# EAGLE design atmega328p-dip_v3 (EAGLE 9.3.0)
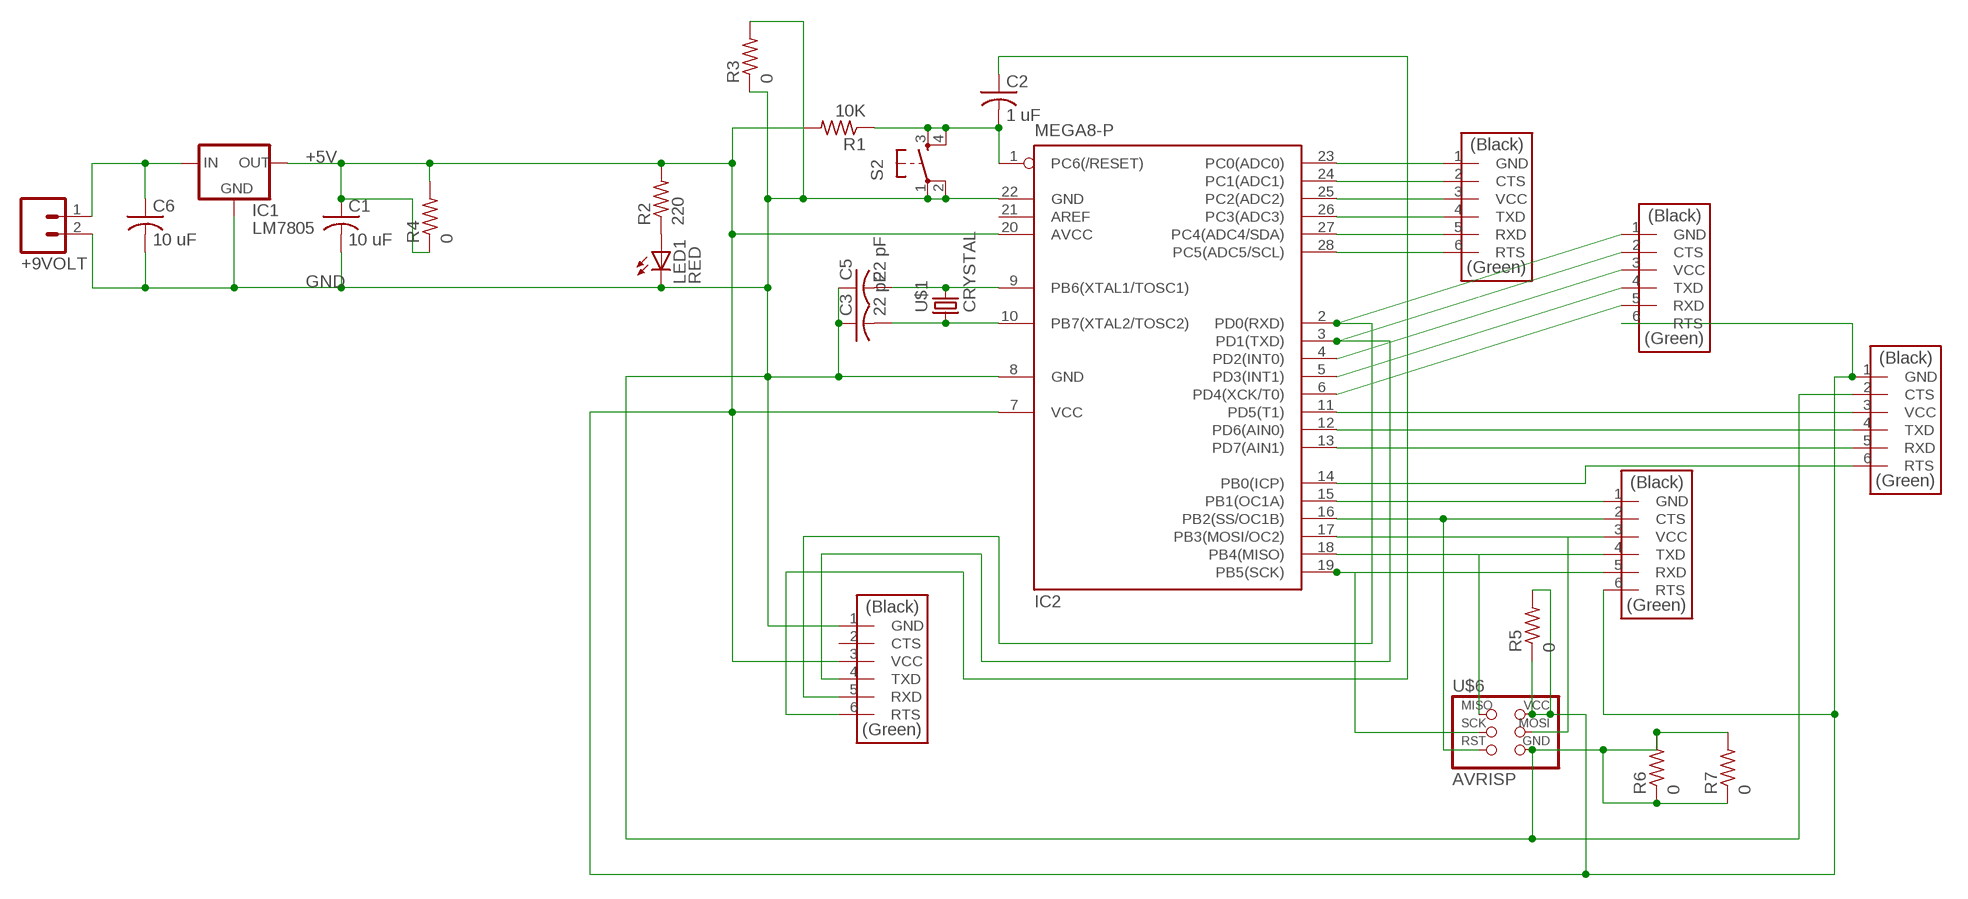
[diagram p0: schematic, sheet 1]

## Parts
+9VOLT  M02PTH4  [1X02_XTRA_BIG]
C1  10 uF  C-USC1206  [C1206]
C2  1 uF  C-USC1206  [C1206]
C3  22 pF  C-USC1206  [C1206]
C5  22 pF  C-USC1206  [C1206]
C6  10 uF  C-USC1206  [C1206]
FTDI  FTDI-SMD-HEADER  [1X06SMD]
IC1  LM7805  V_REG_78XX-TO-220  [TO-220-ALT]
IC2  MEGA8-P  [DIL28-3]
LED1  RED  LEDSMT1206  [1206]
R1  10K  R-US_R1206  [R1206]
R2  220  R-US_R1206  [R1206]
R3  0  R-US_R1206  [R1206]
R4  0  R-US_R1206  [R1206]
R5  0  R-US_R1206  [R1206]
R6  0  R-US_R1206  [R1206]
R7  0  R-US_R1206  [R1206]
S2  6MM_SWITCH6MM_SWITCH  [6MM_SWITCH]
SPIHEADERS  FTDI-SMD-HEADER  [1X06SMD]
U$1  CRYSTAL  [2-SMD-5X3MM]
U$2  FTDI-SMD-HEADER  [1X06SMD]
U$4  FTDI-SMD-HEADER  [1X06SMD]
U$5  FTDI-SMD-HEADER  [1X06SMD]
U$6  AVRISP  [2X03]

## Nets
+5V: C1.1 FTDI.3(VCC) IC1.OUT IC2.7(VCC) IC2.20(AVCC) R1.2 R2.2 R4.1 R4.2 R5.1 R5.2 SPIHEADERS.6(RTS) U$4.6(RTS) U$5.1(GND) U$6.2(VCC)
GND: +9VOLT.2 C1.2 C3.1 C5.1 C6.2 FTDI.1(GND) IC1.GND IC2.8(GND) IC2.22(GND) LED1.C R3.1 R3.2 R6.1 R6.2 R7.1 R7.2 S2.1(P) S2.2(P1) U$5.2(CTS) U$6.6(GND)
N$1: +9VOLT.1 C6.1 IC1.IN
N$3: FTDI.5(RXD) IC2.2(PD0(RXD)) U$4.1(GND)
N$4: LED1.A R2.1
N$5: C5.2 IC2.9(PB6(XTAL1/TOSC1)) U$1.P$2
N$6: C3.2 IC2.10(PB7(XTAL2/TOSC2)) U$1.P$1
N$7: FTDI.4(TXD) IC2.3(PD1(TXD)) U$4.2(CTS)
N$8: C2.1 FTDI.6(RTS)
N$10: C2.2 IC2.1(PC6(/RESET)) R1.1 S2.3(S) S2.4(S1)
N$11: IC2.23(PC0(ADC0)) U$2.1(GND)
N$12: IC2.24(PC1(ADC1)) U$2.2(CTS)
N$13: IC2.25(PC2(ADC2)) U$2.3(VCC)
N$14: IC2.26(PC3(ADC3)) U$2.4(TXD)
N$15: IC2.27(PC4(ADC4/SDA)) U$2.5(RXD)
N$16: IC2.28(PC5(ADC5/SCL)) U$2.6(RTS)
N$17: IC2.4(PD2(INT0)) U$4.3(VCC)
N$18: IC2.5(PD3(INT1)) U$4.4(TXD)
N$19: IC2.6(PD4(XCK/T0)) U$4.5(RXD)
N$20: IC2.15(PB1(OC1A)) SPIHEADERS.1(GND)
N$21: IC2.16(PB2(SS/OC1B)) SPIHEADERS.2(CTS) U$6.5(RST)
N$22: IC2.17(PB3(MOSI/OC2)) SPIHEADERS.3(VCC) U$6.4(MOSI)
N$23: IC2.18(PB4(MISO)) SPIHEADERS.4(TXD) U$6.1(MISO)
N$24: IC2.19(PB5(SCK)) SPIHEADERS.5(RXD) U$6.3(SCK)
N$25: IC2.11(PD5(T1)) U$5.3(VCC)
N$26: IC2.12(PD6(AIN0)) U$5.4(TXD)
N$27: IC2.13(PD7(AIN1)) U$5.5(RXD)
N$28: IC2.14(PB0(ICP)) U$5.6(RTS)
Unconnected: FTDI.2(CTS) IC2.21(AREF)

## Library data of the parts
+9VOLT = SparkFun:M02: Header 2
C1-C3 C5 C6 = adafruit:C-US: CAPACITOR, American symbol
FTDI SPIHEADERS U$2 U$4 U$5 = fab:FTDI-SMD-HEADER
IC1 = SparkFun:V_REG_78XX: Voltage Regulator Standard 7805 5V regulator. IGO (Input Ground Output). Spark Fun Electronics SKU : COM-00107
IC2 = atmel:MEGA8-P: MICROCONTROLLER 8 Kbytes FLASH, 1 kbytes SRAM, 512 bytes EEPROM, USART, 4-channel 10 bit ADC, 2-channel 8 bit ADC Pin compatible with Atmega48, ATMega88, ATMega168 Source: avr.lbr; OC_FARNELL: unknown; OC_NEWARK: unknown
LED1 = adafruit:LED: LED
R1-R7 = rcl:R-US_: RESISTOR, American symbol; SPICEPREFIX: R
S2 = fab:6MM_SWITCH: OMRON SWITCH
U$1 = fab:CRYSTAL
U$6 = fab:AVRISP

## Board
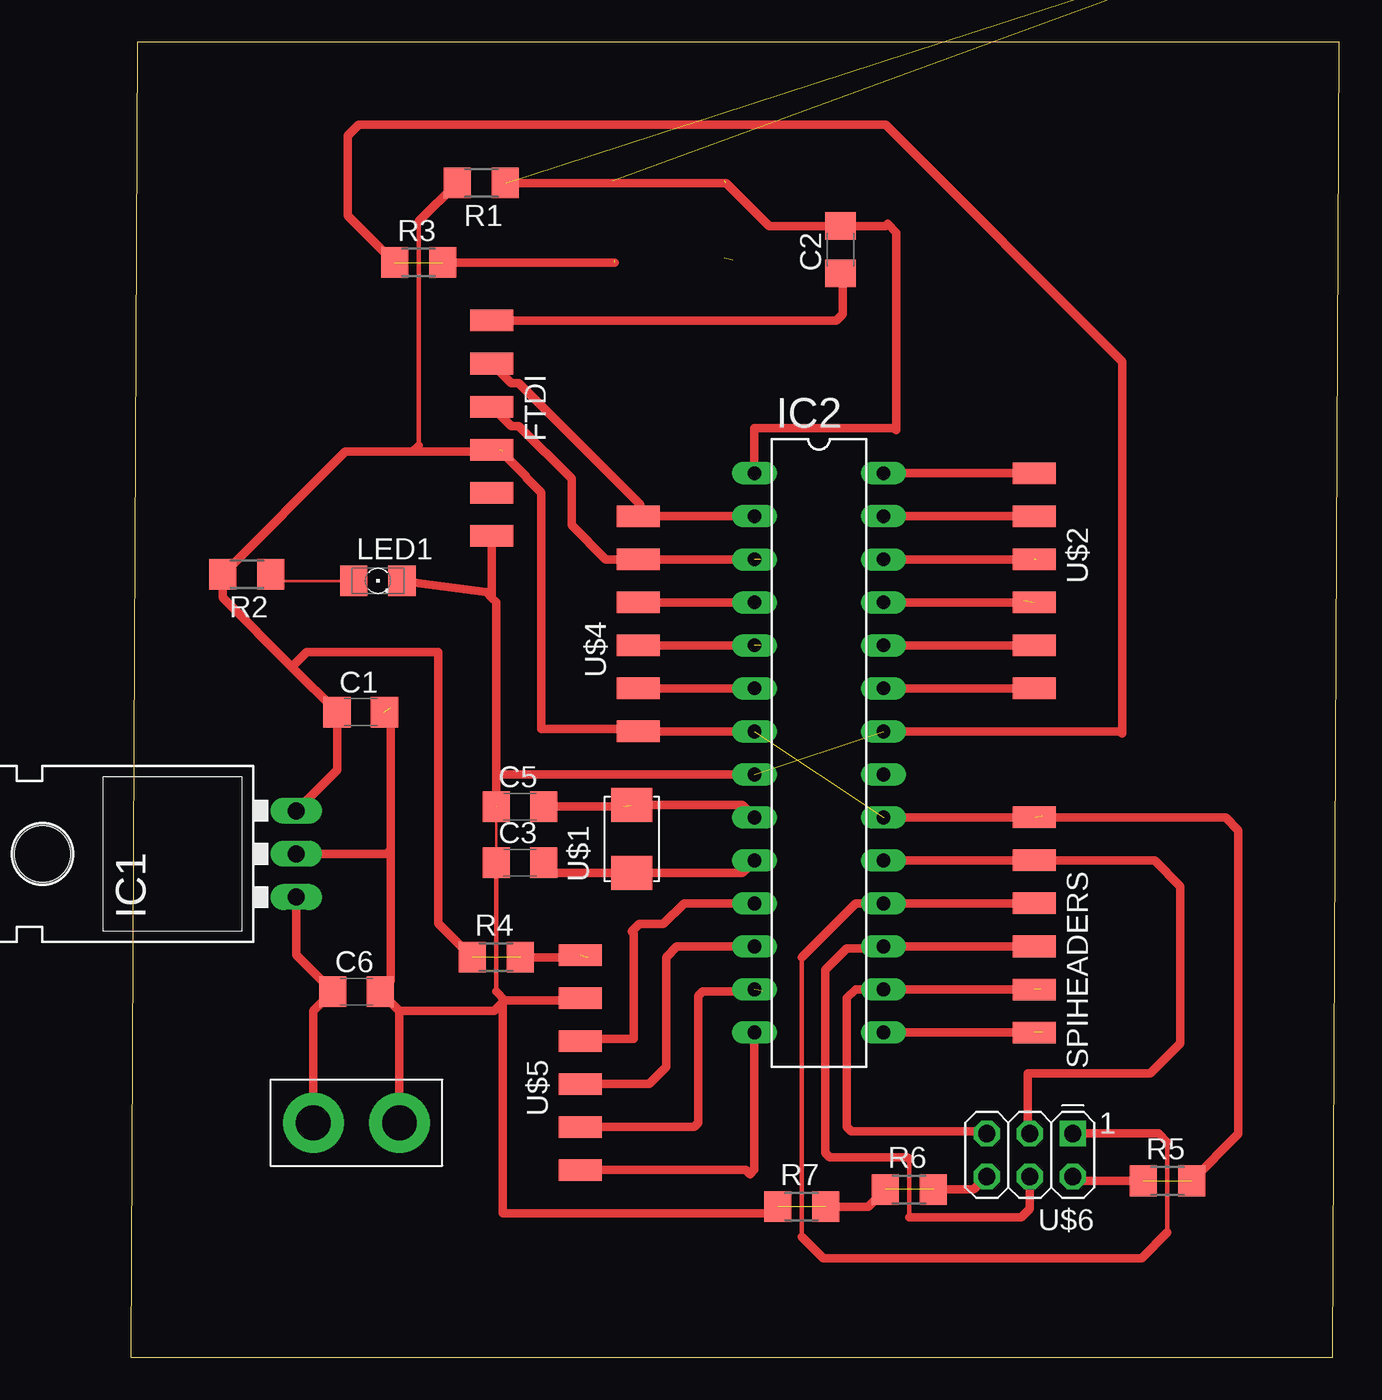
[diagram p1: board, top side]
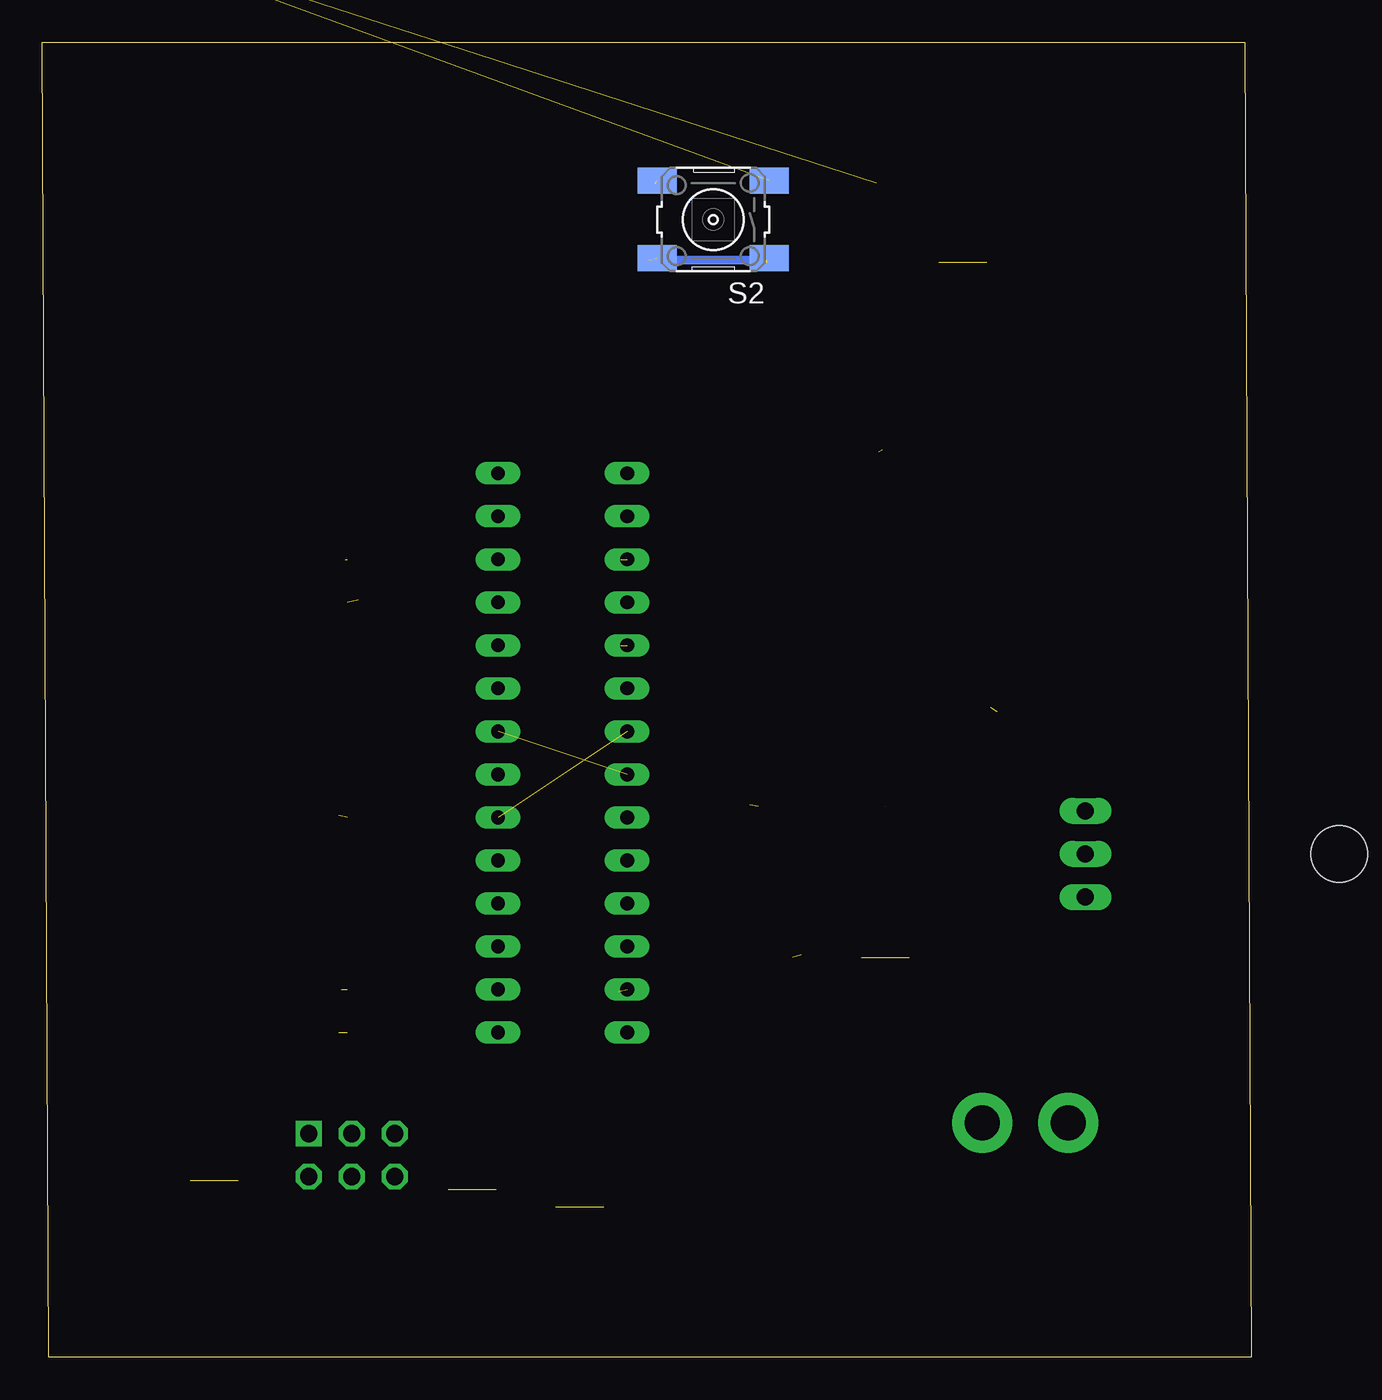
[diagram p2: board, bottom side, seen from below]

Size 71.35 x 77.65 mm. Coordinates in mm from the lower left corner, seen from the top.
Outline: 0,0 70.97,0 71.35,77.65 0.38,77.65 0,0
Copper layers (1*16): Top 0.035mm / dielectric 1.5mm / Bottom 0.035mm
Design rules "default *": minimum track width 20mil, minimum drill 0.35mm, track to track 20mil, track to pad 20mil, pad to pad 20mil, via to via 20mil, smd to smd 20mil, copper to edge 40mil, drill to drill 6mil, minimum pad ring 10mil, minimum via ring 8mil, stop-mask expansion 4mil, vias tented up to drill 0mil, thermal gap 10mil

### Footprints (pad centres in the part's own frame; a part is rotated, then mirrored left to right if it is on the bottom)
1X02_XTRA_BIG = drill 2.057 pad 3.556: 1 -2.54,0; 2 2.54,0
C1206 = smd 1.6 x 1.8: 1 -1.4,0; 2 1.4,0
1X06SMD = smd 2.54 x 1.27: 1 0,6.35; 2 0,3.81; 3 0,1.27; 4 0,-1.27; 5 0,-3.81; 6 0,-6.35
TO-220-ALT = drill 1.016 long: GND 0,-3.81; IN -2.54,-3.81; OUT 2.54,-3.81 | hole 3.302: 0,11.176
DIL28-3 = drill 0.813 long: 1 -16.51,-3.81; 2 -13.97,-3.81; 3 -11.43,-3.81; 4 -8.89,-3.81; 5 -6.35,-3.81; 6 -3.81,-3.81; 7 -1.27,-3.81; 8 1.27,-3.81; 9 3.81,-3.81; 10 6.35,-3.81; 11 8.89,-3.81; 12 11.43,-3.81; 13 13.97,-3.81; 14 16.51,-3.81; 15 16.51,3.81; 16 13.97,3.81; 17 11.43,3.81; 18 8.89,3.81; 19 6.35,3.81; 20 3.81,3.81; 21 1.27,3.81; 22 -1.27,3.81; 23 -3.81,3.81; 24 -6.35,3.81; 25 -8.89,3.81; 26 -11.43,3.81; 27 -13.97,3.81; 28 -16.51,3.81
1206 = smd 1.6 x 1.803: A -1.422,0; C 1.422,0
R1206 = smd 1.6 x 1.803: 1 -1.422,0; 2 1.422,0
6MM_SWITCH = smd 2.286 x 1.524: 1 -3.302,2.286; 2 3.302,2.286; 3 -3.302,-2.286; 4 3.302,-2.286
2-SMD-5X3MM = smd 2 x 2.4: P$1 -2,0; P$2 2,0
2X03 = drill 1.016 square: 1 -2.54,-1.27 | drill 1.016 octagon: 2 -2.54,1.27; 3 0,-1.27; 4 0,1.27; 5 2.54,-1.27; 6 2.54,1.27

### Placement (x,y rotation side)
+9VOLT  13.34,13.84 0 top
C1  13.59,38.1 0 top
C2  41.91,65.41 90 top
C3  22.99,29.21 0 top
C5  22.99,32.51 0 top
C6  13.34,21.59 0 top
FTDI  21.34,54.86 180 top
IC1  5.97,29.72 90 top
IC2  40.64,35.69 270 top
LED1  14.61,45.85 0 top
R1  20.7,69.34 180 top
R2  6.86,46.23 180 top
R3  17.02,64.64 0 top
R4  21.59,23.62 0 top
R5  61.21,10.41 0 top
R6  45.97,9.91 0 top
R7  39.62,8.89 0 top
S2  31.75,67.18 180 bottom
SPIHEADERS  53.34,25.53 180 top
U$1  29.59,30.61 90 top
U$2  53.34,45.85 180 top
U$4  29.97,43.31 0 top
U$5  26.54,17.4 0 top
U$6  53.09,11.94 180 top

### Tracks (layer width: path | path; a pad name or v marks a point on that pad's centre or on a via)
+5V  (6 unrouted)
  Top 0.152: 6.58,47.37 R2.2
  Top 0.254: 17.02,67.08 17.02,53.85
  Top 0.508: 16.64,53.47 12.68,53.47 R2.2 5.44,44.85 9.52,40.77 | 16.64,53.47 21.97,53.47 | R1.2 17.02,67.08 | 17.02,53.85 16.64,53.47 | IC2.7 U$4.6 29.84,37.08 24.26,37.08 24.26,51.05 23.37,51.94 23.37,52.01 21.78,53.59 FTDI.3 | IC2.20 SPIHEADERS.6 64.64,31.88 65.41,31.11 65.41,13.18 R5.2 | IC1.OUT 12.19,34.67 C1.1 9.52,40.77 | R4.2 27.05,23.62 | R4.1 18.16,25.63 18.16,41.66 10.41,41.66 9.52,40.77 | 54.1,31.75 53.85,32 | U$6.2 55.88,10.41 R5.1
GND  (8 unrouted)
  Top 0.152: +9VOLT.2 15.99,13.96 | C3.1 21.59,32.13 C5.1 22.1,33.02
  Top 0.254: C3.1 21.59,21.59
  Top 0.508: 21.59,21.59 22.1,21.08 | 22.1,21.08 26.42,21.08 U$5.2 | IC2.8 21.84,34.42 21.59,34.16 21.59,32.13 | LED1.C 20.99,45.18 21.34,44.83 | 21.34,44.83 FTDI.1 | C5.1 21.59,44.58 21.34,44.83 | IC2.22 58.42,36.96 58.55,36.83 58.55,58.8 44.58,72.77 13.46,72.77 12.83,72.14 12.83,67.41 R3.1 | +9VOLT.2 15.88,20.45 | 15.88,20.45 C6.2 15.37,22.22 15.37,29.97 | 15.37,29.97 15.37,38.35 | IC1.GND 15.11,29.72 15.37,29.97 | 15.88,20.45 21.47,20.45 21.97,20.95 | R3.2 28.57,64.64 | 22.1,21.08 21.97,20.95 | 21.97,20.95 21.97,8.51 37.82,8.51 R7.1 | R6.2 49.78,9.91 U$6.6 | R7.2 43.54,8.89 R6.1
  Bottom 0.508: S2.1 28.57,64.77 35.56,64.77
N$1
  Top 0.152: +9VOLT.1 10.65,14.32
  Top 0.508: +9VOLT.1 10.79,20.45 C6.1 9.78,23.75 IC1.IN
N$3
  Top 0.508: U$4.1 30.1,49.66 | 30.1,49.66 IC2.2 | FTDI.5 22.48,57.53 22.92,57.53 30.1,50.35 30.1,49.66
N$4
  Top 0.152: LED1.A 8.98,45.85 R2.1
N$5  (1 unrouted)
  Top 0.508: U$1.P$2 36.1,32.61 IC2.9 | C5.2 29.08,32.51
N$6
  Top 0.508: IC2.10 36.1,28.61 U$1.P$1 24.99,28.61 C3.2
N$7  (1 unrouted)
  Top 0.508: 37.47,46.86 37.21,47.12 U$4.2 28.07,47.12 26.04,49.15 26.04,51.88 22.92,54.99 22.48,54.99 FTDI.4
N$8
  Top 0.508: FTDI.6 41.66,61.21 42.04,61.59 42.04,63.88 C2.1
N$10  (3 unrouted)
  Top 0.508: 22.5,69.72 R1.1 35.18,69.34 37.72,66.81 C2.2 44.58,66.81 44.7,66.93 45.21,66.42 45.21,54.74 45.09,54.86 36.83,54.86 IC2.1
N$11
  Top 0.508: IC2.23 U$2.1
N$12
  Top 0.508: IC2.24 U$2.2
N$13  (1 unrouted)
  Top 0.508: IC2.25 52.58,44.58 52.7,44.7
N$14  (1 unrouted)
  Top 0.508: IC2.26 53.47,47.12 53.85,46.74
N$15
  Top 0.508: IC2.27 U$2.5
N$16
  Top 0.508: IC2.28 U$2.6
N$17
  Top 0.508: U$4.3 IC2.4
N$18  (1 unrouted)
  Top 0.508: U$4.4 37.21,42.04 37.47,42.29
N$19
  Top 0.508: U$4.5 IC2.6
N$20  (1 unrouted)
  Top 0.508: IC2.15 53.85,19.18 53.98,19.05
N$21  (1 unrouted)
  Top 0.508: 53.85,21.84 53.72,21.72 IC2.16 42.8,21.72 42.29,21.21 42.29,13.59 42.55,13.34 50.42,13.34 U$6.5
N$22
  Top 0.254: 45.97,11.68 45.97,8.26
  Top 0.508: SPIHEADERS.3 IC2.17 44.32,24.13 42.29,24.13 41.02,22.86 41.02,12.06 41.27,11.81 45.85,11.81 45.97,11.68 | 52.83,10.41 U$6.4 53.09,8.76 52.58,8.26 45.97,8.26
N$23
  Top 0.254: 39.62,23.62 39.62,7.11 | 61.21,7.37 61.21,12.7
  Top 0.508: SPIHEADERS.4 IC2.18 42.8,26.8 39.62,23.62 | 39.62,7.11 40.89,5.84 59.69,5.84 61.21,7.37 | U$6.1 60.71,13.21 61.21,12.7
N$24
  Top 0.508: IC2.19 SPIHEADERS.5 60.45,29.34 61.98,27.81 61.98,18.54 60.2,16.76 52.96,16.76 52.96,13.34 U$6.3
N$25
  Top 0.508: U$5.3 26.67,18.8 29.72,18.8 29.72,25.02 29.59,25.15 30.02,25.57 31.46,25.57 32.68,26.8 IC2.11
N$26
  Top 0.508: U$5.4 30.61,16.13 31.62,17.14 31.62,23.62 32.26,24.26 IC2.12
N$27  (1 unrouted)
  Top 0.508: U$5.5 33.27,13.59 33.53,13.84 33.53,21.34 33.78,21.59 37.34,21.59 37.47,21.72
N$28
  Top 0.508: U$5.6 36.32,11.05 36.58,10.79 36.83,11.05 IC2.14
